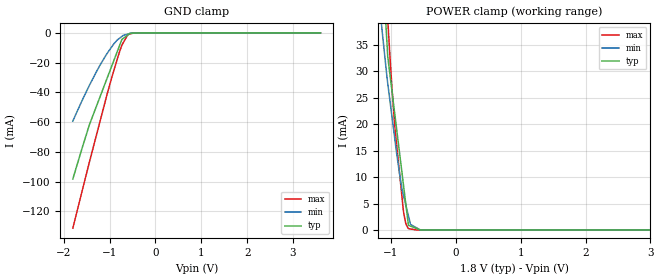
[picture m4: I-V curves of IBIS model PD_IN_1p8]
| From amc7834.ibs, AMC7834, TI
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|   Model
[Model]   PD_IN_1p8
Model_type   Input
Vinl = 0.54
Vinh = 1.26
|   typ   min   max
C_comp   9.202pF   6.403pF   9.427pF
[Voltage Range]   1.8   1.7   1.9
[Temperature Range]   27   125   -40
[Power Clamp Reference]   1.8   1.7   1.9
[GND Clamp Reference]   0   0   0
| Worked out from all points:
|   GND clamp passes 1 mA (typ) near -0.58 V on its own axis
|   POWER clamp passes 1 mA (typ) near -0.73 V on its own axis
[GND Clamp]
|   Voltage   I(typ)   I(min)   I(max)
-1.8V     -98.23mA   -59.33mA   -131.3mA
-1.438V   -61.71mA   -35.22mA   -86.82mA
-1.19V    -41.58mA   -20.77mA   -57.44mA
-968.4mV  -23.64mA   -10.11mA   -31.88mA
-828mV    -12.27mA   -4.676mA   -17.28mA
-730.8mV  -4.392mA   -2.389mA   -8.279mA
-601.2mV  -1.421mA   -773.4uA   -1.147mA
-547.2mV  -183.3uA   -299.5uA   -682.2uA
-471.6mV  -119.8uA   -102.2uA   -30.83uA
-266.4mV  -6.796nA   -769nA     0A
3.6V      0A         0A         0A
[POWER Clamp]
|   Voltage   I(typ)   I(min)   I(max)
-1.8V     205.6mA    162.9mA    239.3mA
-1.19V    62.6mA     43.95mA    75.48mA
-1.06V    35.06mA    28.73mA    42.24mA
-1.039V   31.67mA    26.64mA    37.54mA
-984.6mV  26.27mA    21.44mA    26.91mA
-936mV    21.41mA    16.76mA    18.87mA
-807.9mV  8.589mA    6.579mA    3.618mA
-768.6mV  4.663mA    4.59mA     1.17mA
-730.8mV  882.6uA    2.676mA    248uA
-698.4mV  727uA      1.035mA    186.2uA
-547.2mV  994nA      19.14uA    274.6nA
3.6V      0A         0A         0A
